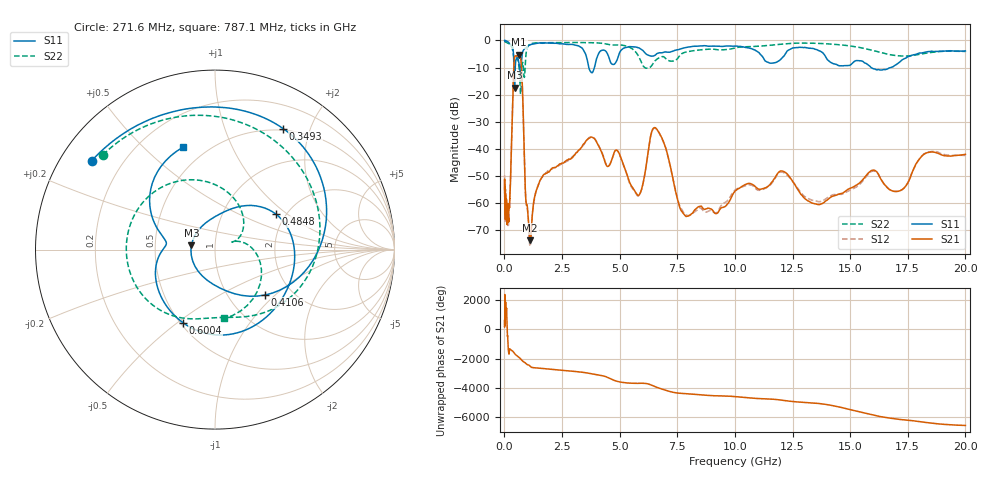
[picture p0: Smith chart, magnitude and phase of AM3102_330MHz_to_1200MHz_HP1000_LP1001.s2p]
! Date/Time: Tue, Sep 11, 2018 5:17 PM
! Network Analyzer: Agilent Technologies E8362B Rev: A.07.50.63
! Sweep from 0.010 to 20.000 GHz, 1601 Points, Sweep Type: LOG
! Power Supply: 4.949 V, 0.001 A
# Hz S DB R 50
!freq MagS11 AngS11 MagS21 AngS21 MagS12 AngS12 MagS22 AngS22
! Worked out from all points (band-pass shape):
!   1601 points, 10 MHz to 20 GHz, reference 50 ohm
!   highest |S21| = -5.27 dB at 632.6 MHz (marker M1); lowest = -73.7 dB at 1.124 GHz (marker M2)
!   |S21| within 3 dB of the highest: 419 MHz to 727.8 MHz (308.8 MHz wide, 53.8 % of centre)
!   lowest |S11| = -17.5 dB at 440.9 MHz (marker M3), VSWR 1.31, Z = 38.4 + j1.95 ohm
!   |S11| at or under -10 dB: 661.3 MHz to 720 MHz (58.72 MHz wide, 8.5 % of centre); 3.663 GHz to 3.907 GHz (243.1 MHz wide, 6.42 % of centre); 15.91 GHz to 16.76 GHz (850.4 MHz wide, 5.21 % of centre)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
!   |S22| runs from -19.7 to -0.2 dB; largest |S21 - S12| = 0.01
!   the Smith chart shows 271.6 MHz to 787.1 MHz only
!   S11 on the Smith chart (normalised r, x): 271.6 MHz: 0.09, +0.32; 349.3 MHz: 0.48, +1.61; 410.6 MHz: 1.47, -0.87; 484.8 MHz: 1.77, +0.83; 600.4 MHz: 0.52, -0.52; 787.1 MHz: 0.37, +0.66
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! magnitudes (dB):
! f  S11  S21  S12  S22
! 10 MHz  0.0  -55.1  -49.8  -0.2
! 35.55 MHz  0.0  -61.4  -63.4  -0.4
! 126.4 MHz  -0.4  -65.7  -65.0  -0.9
! 177.9 MHz  -0.7  -65.8  -67.4  -1.1
! 271.6 MHz  -1.4  -50.1  -50.0  -1.7
! 349.3 MHz  -2.2  -26.1  -26.2  -3.2
! 410.6 MHz  -8.5  -9.6  -9.7  -6.7
! 440.9 MHz  -17.5  -6.2  -6.3  -8.4
! 447.2 MHz  -17.0  -6.0  -6.0  -8.4
! 484.8 MHz  -8.1  -5.7  -5.7  -6.8
! 600.4 MHz  -7.0  -5.4  -5.6  -7.6
! 632.6 MHz  -8.4  -5.3  -5.3  -9.8
! 705.6 MHz  -11.0  -6.6  -6.6  -19.7
! 787.1 MHz  -4.5  -18.6  -18.7  -8.2
! 920.7 MHz  -2.8  -57.4  -57.7  -6.9
! 1.124 GHz  -1.6  -73.7  -75.8  -1.3
! 1.59 GHz  -1.0  -51.1  -51.0  -0.8
! 3.775 GHz  -11.9  -35.7  -35.6  -0.8
! 5.652 GHz  -2.4  -55.4  -55.7  -3.8
! 6.58 GHz  -5.1  -32.5  -32.6  -7.2
! 7.92 GHz  -2.5  -64.9  -64.5  -4.2
! 20 GHz  -3.9  -42.1  -42.5  -4.1
